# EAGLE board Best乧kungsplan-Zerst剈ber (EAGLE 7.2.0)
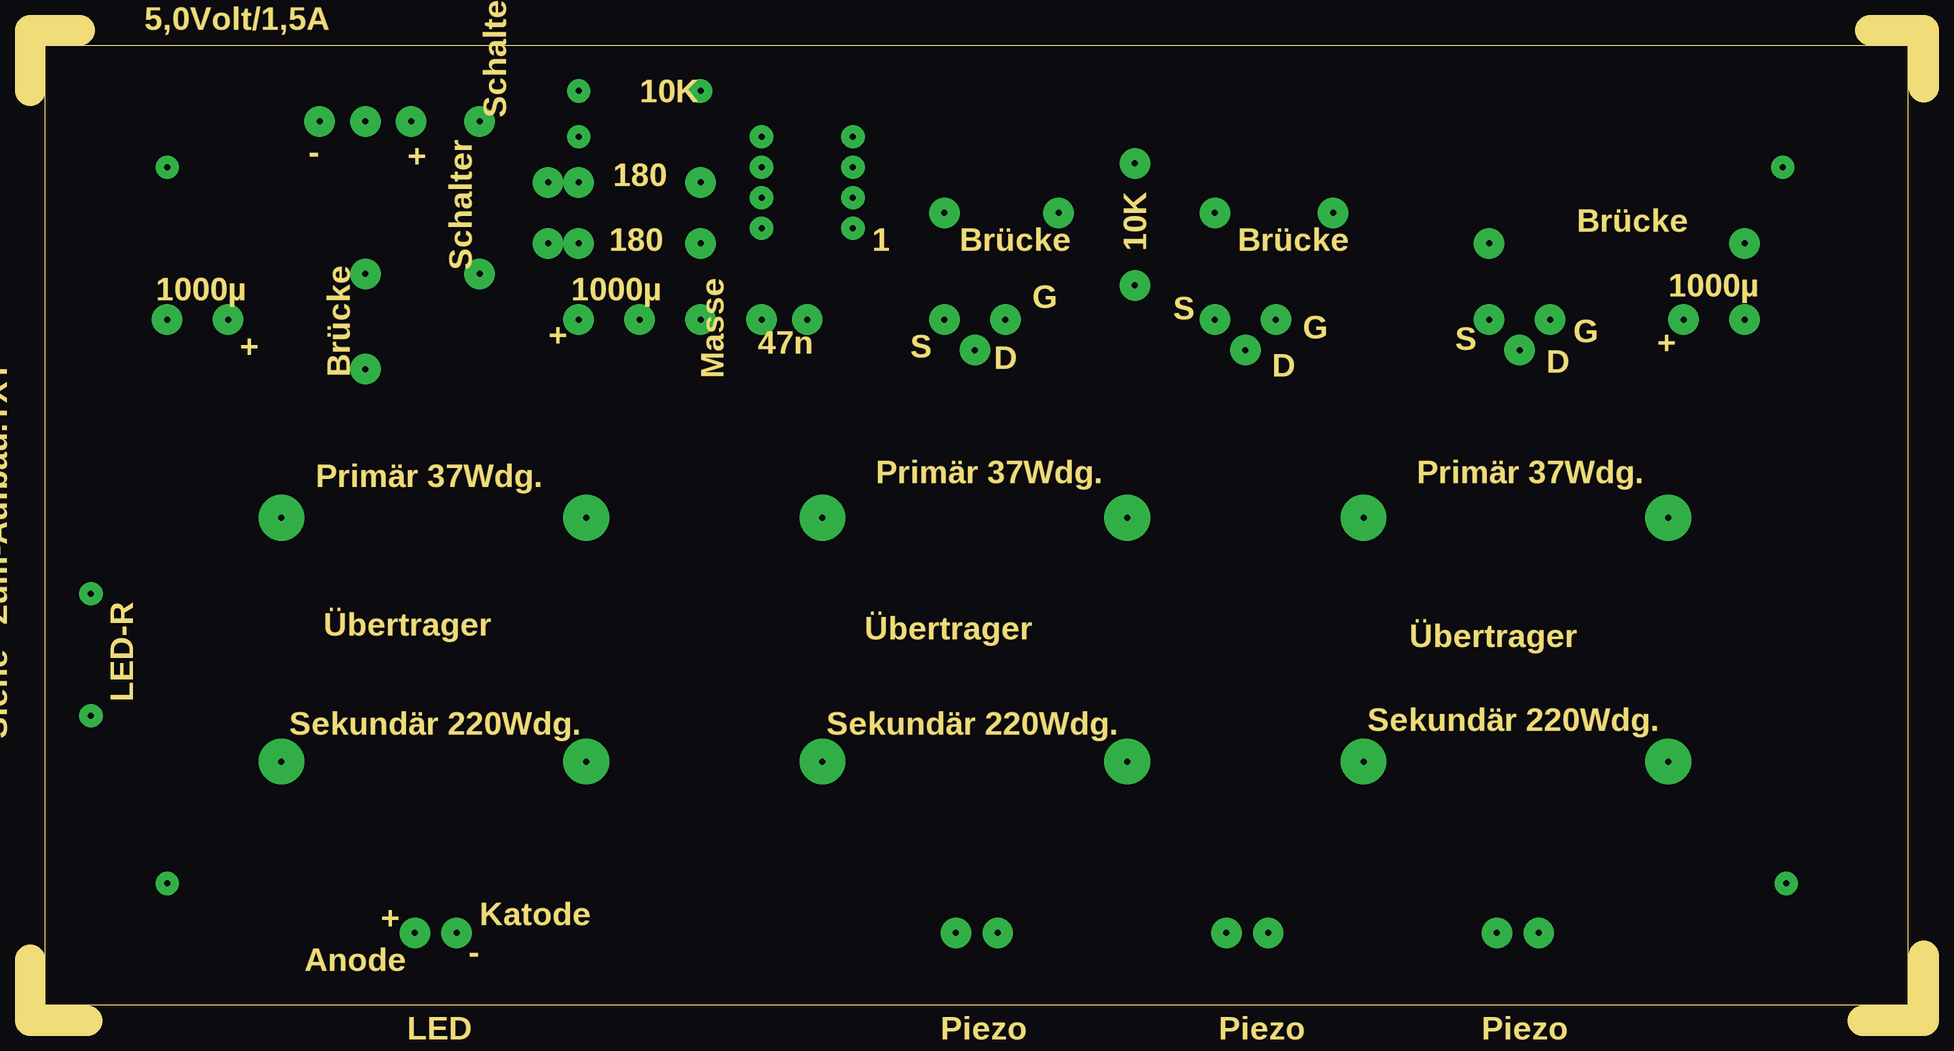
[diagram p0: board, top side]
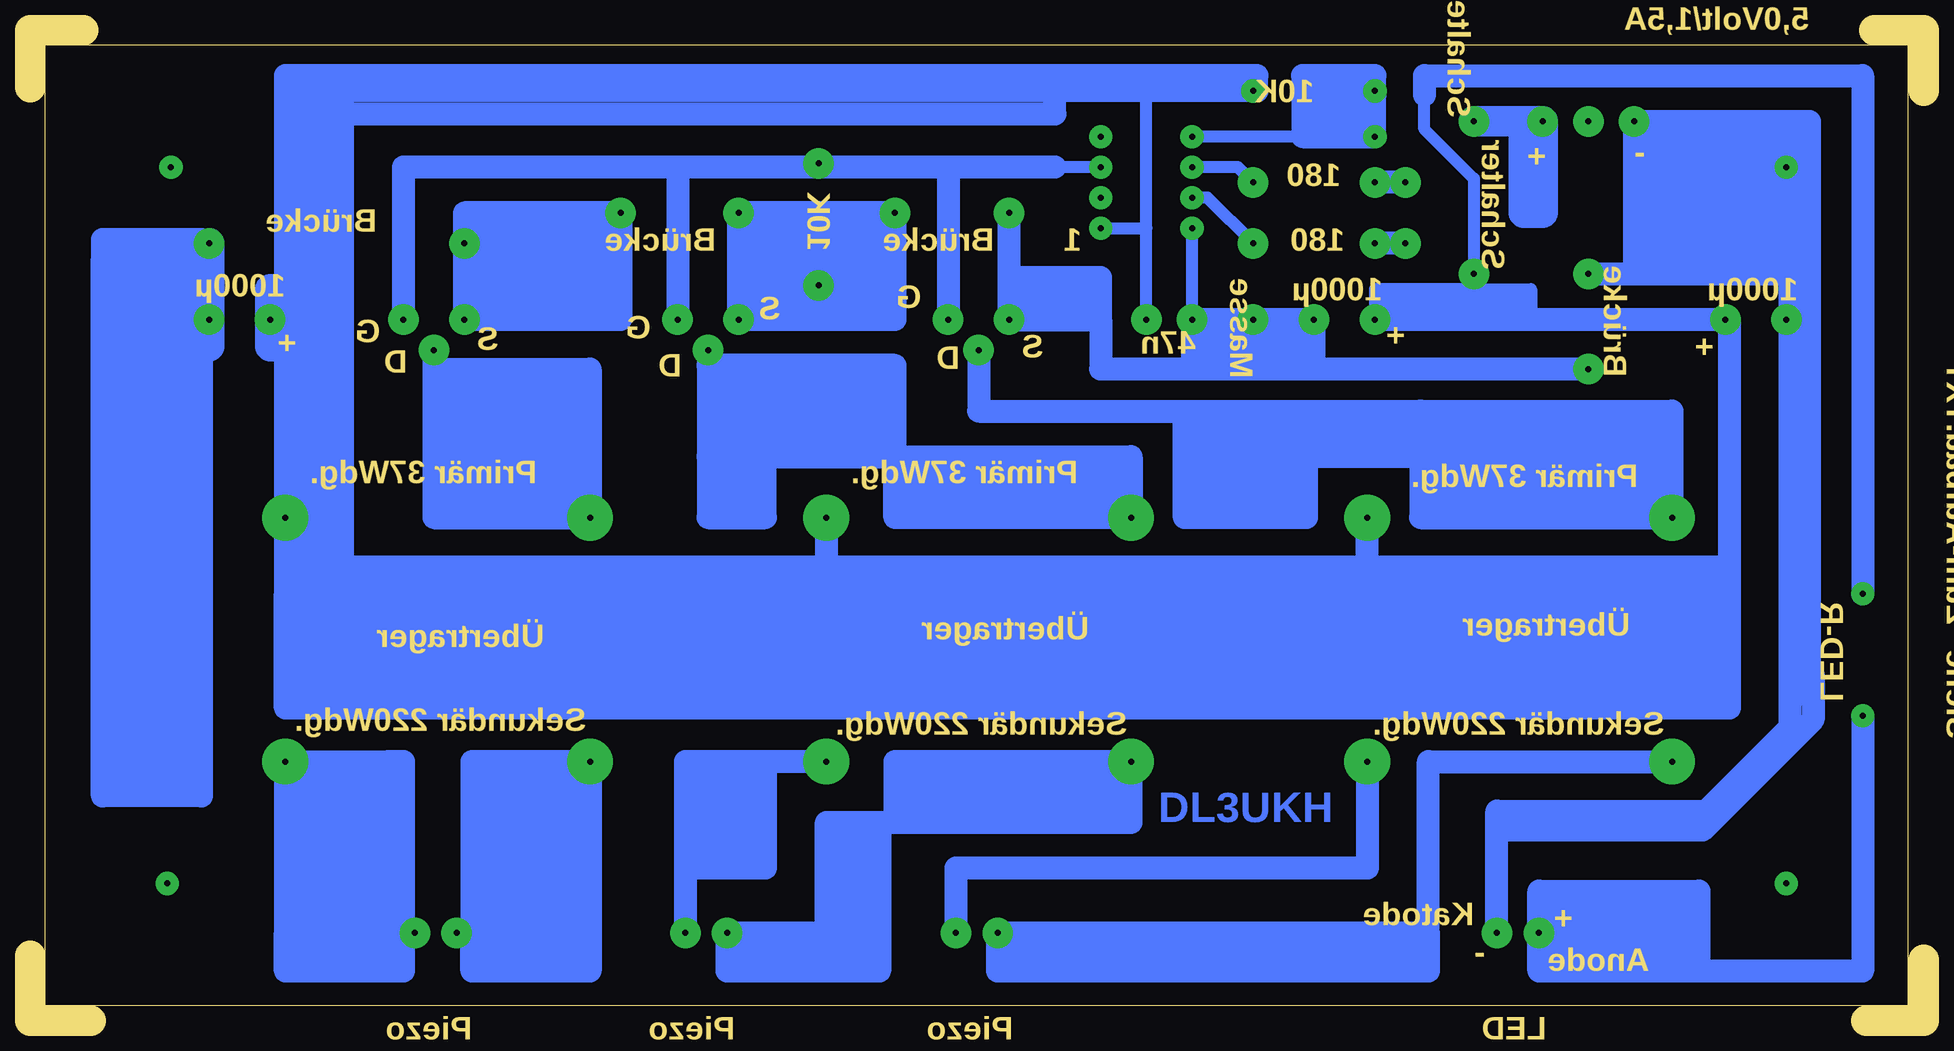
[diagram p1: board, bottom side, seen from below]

Size 157.8 x 82.55 mm. Coordinates in mm from the lower left corner, seen from the top.
Outline: 157.8,5.4 157.8,0.32
Outline: 157.8,0 152.72,0
Outline: 157.8,77.79 157.8,82.55 153.35,82.55
Outline: 0,5.08 0,0 4.76,0
Outline: 4.13,82.55 0,82.55
Outline: 0,77.47 0,82.23
Outline: 156.53,1.27 156.53,81.28 1.27,81.28 1.27,1.27 156.53,1.27
Copper layers (1*16): Top 0.035mm / dielectric 1.5mm / Bottom 0.035mm
Design rules "default": minimum track width 10mil, minimum drill 24mil, track to track 8mil, track to pad 8mil, pad to pad 8mil, via to via 8mil, smd to smd 8mil, copper to edge 40mil, drill to drill 8mil, minimum pad ring 10mil, minimum via ring 8mil, stop-mask expansion 4mil, vias tented up to drill 0mil, thermal gap 10mil

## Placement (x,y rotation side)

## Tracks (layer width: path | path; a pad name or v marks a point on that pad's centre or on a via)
S$1  (via drill 0.5 pad 1.93)
  other vias: 11.43,71.12
S$2  (via drill 0.5 pad 1.93)
  other vias: 11.43,11.43
S$3  (via drill 0.5 pad 1.93)
  other vias: 146.05,71.12
S$4  (via drill 0.5 pad 1.93)
  other vias: 146.37,11.43
S$5  (via drill 0.5 pad 1.93)
  other vias: 5.08,35.56
S$6  (via drill 0.5 pad 2.54)
  Bottom 1.016: 11.11,61.6 11.43,62.23 14.92,62.23
  Bottom 1.93: v35.56,7.3 35.56,17.46 18.1,17.46 11.11,24.45 11.11,61.6 11.11,62.23 | 27.94,62.23 24.13,62.23 | 24.13,62.23 11.43,62.23 | 14.92,74.93 v24.13,74.93 24.13,62.23 | 14.92,74.93 14.92,62.23 | 14.92,74.93 9.53,74.93 9.53,61.91 | 9.53,61.91 14.29,62.87 14.61,62.23 | 9.53,61.91 9.53,26.99
S$7  (via drill 0.5 pad 2.54)
  Bottom 1.016: v60.96,58.42 60.96,66.04 | 55.88,54.61 55.88,53.98 | 60.96,53.98 60.96,54.61 | 55.88,53.98 60.96,53.98 | 50.8,53.98 55.88,53.98 | 50.8,54.93 50.8,53.98 | 27.62,53.98 50.8,53.98 | 60.96,53.98 68.58,53.98 68.58,54.29
  Bottom 1.93: v55.88,58.42 55.88,54.61 | 50.8,54.93 v50.8,58.42 v60.96,58.42 60.96,54.61 | 76.2,61.91 v76.2,58.42 68.58,58.42 | 76.2,61.91 v76.2,67.31 | 68.58,58.42 68.58,54.29 v27.94,54.29 | 68.58,58.42 68.58,61.91 76.2,61.91
S$8  (via drill 0.5 pad 2.54)
  Bottom 1.93: v43.18,69.85 v45.72,69.85
S$9  (via drill 0.5 pad 2.54)
  Bottom 1.93: v43.18,64.77 v45.72,64.77
S$10  (via drill 0.5 pad 2.54, 0.5 pad 3.81)
  Bottom 1.93: v99.69,7.3 91.44,7.3 | 91.44,7.3 91.44,16.51 86.99,16.51 | 86.99,16.51 85.72,16.51 | 85.72,16.51 66.04,16.51 v66.04,21.59 85.72,21.59 85.72,16.51 | 91.44,7.3 91.44,4.13 | 91.44,4.13 92.08,4.13 99.69,4.13 99.69,6.98 | 86.99,16.51 86.99,4.13 91.44,4.13
S$11  (via drill 0.5 pad 2.54)
  Bottom 1.93: v85.72,67.31 85.72,58.42 v98.74,58.42 v98.74,67.31 v85.72,67.31
S$12  (via drill 0.5 pad 2.54, 0.5 pad 3.81)
  Bottom 1.93: v78.74,55.88 78.74,50.8 41.91,50.8 | 41.91,50.8 20.95,50.8 v20.95,41.91 41.91,41.91 41.91,46.99 | 41.91,50.8 41.91,46.99 | 41.91,46.99 51.44,46.99 | 51.44,46.99 61.6,46.99 | 61.6,46.99 61.6,47.31 61.6,50.48 | 51.44,46.99 51.44,41.91 61.6,41.91 61.6,46.99
S$13  (via drill 0.5 pad 2.54)
  Bottom 1.93: 33.02,74.93 33.34,74.93
  Bottom 2.54: v37.47,74.93 33.34,74.93 33.34,67.31 31.75,67.31 v31.75,74.93 33.02,74.93
S$14  (via drill 0.5 pad 2.54, 0.5 pad 3.81)
  Bottom 1.93: v46.36,21.59 46.36,12.7 80.64,12.7 v80.64,7.3
S$15  (via drill 0.5 pad 2.54)
  other vias: 27.94,62.23
S$16  (via drill 0.5 pad 2.54)
  Bottom 1.93: v108.58,67.31 108.58,58.42 v121.6,58.42 v121.6,64.77 121.6,67.31 v108.58,67.31
S$17  (via drill 0.5 pad 2.54, 0.5 pad 3.81)
  Bottom 1.93: 41.28,7.3 v77.15,7.3 77.15,4.13 41.28,4.13 41.28,7.3 | 41.28,7.3 41.28,21.59 v20.95,21.59
S$18  (via drill 0.5 pad 2.54, 0.5 pad 3.81)
  Bottom 1.93: v91.44,21.59 96.52,21.59 | 96.52,21.59 103.19,21.59 v103.19,7.3 | 96.52,21.59 96.52,12.7 102.87,12.7
S$19  (via drill 0.5 pad 2.54)
  other vias: 11.43,58.42
S$20  (via drill 0.5 pad 2.54)
  other vias: 27.94,74.93
S$21  (via drill 0.5 pad 1.93)
  Bottom 1.016: v45.72,77.47 52.07,77.47 52.07,73.66 | 52.07,73.66 v60.96,73.66 | 51.75,73.66 52.07,73.66
  Bottom 1.93: v45.72,77.47 45.72,78.74 51.75,78.74 51.75,73.66 v45.72,73.66 45.72,77.15 v45.72,77.47
S$22  (via drill 0.5 pad 2.54, 0.5 pad 3.81)
  Bottom 1.93: 136.53,7.3 v136.53,21.59 127.95,21.59 | 136.53,7.3 v125.73,7.3 | 126.68,4.13 136.53,4.13 136.53,7.3 | 127.95,21.59 127.95,6.67 | 126.68,21.59 127.95,21.59
S$23  (via drill 0.5 pad 1.93, 0.5 pad 2.54)
  Bottom 1.016: v55.88,69.85 57.15,71.12 v60.96,71.12
S$24  (via drill 0.5 pad 1.93, 0.5 pad 2.54)
  Bottom 1.93: v5.08,25.4 5.08,4.13 18.73,4.13 | 18.73,4.13 32.07,4.13 v32.07,7.3 | v32.07,7.3 18.73,7.3 | 18.73,7.3 18.73,6.98 18.73,4.13 | v32.07,7.3 32.07,10.79 18.73,10.79 18.73,7.3
S$25  (via drill 0.5 pad 2.54)
  other vias: 92.08,71.44
S$26  (via drill 0.5 pad 1.93, 0.5 pad 2.54)
  Bottom 1.016: v55.88,64.77 59.69,68.58 v60.96,68.58
S$27
  Bottom 1.93: 131.45,75.56 72.39,75.56 72.39,77.15
S$28  (via drill 0.5 pad 2.54)
  other vias: 92.08,61.28
S$29  (via drill 0.5 pad 2.54, 0.5 pad 3.81)
  Bottom 1.93: v124.14,55.88 124.14,54.29 | 124.14,54.29 124.14,41.91 v111.12,41.91 111.12,54.29 124.14,54.29
S$30
  Bottom 1.93: 9.21,28.89 9.21,25.08 18.41,15.88 35.24,15.88
S$31
  Bottom 1.93: 143.51,63.5 143.51,18.73 151.77,18.73 151.77,63.18 151.77,63.5 | 151.77,63.5 143.51,63.5 | 143.51,63.5 143.51,65.09 151.77,65.09 151.77,63.5
S$32  (via drill 0.5 pad 2.54, 0.5 pad 3.81)
  Bottom 1.93: v101.28,55.88 101.28,54.61 | 101.28,54.61 101.28,46.99 | 101.28,46.99 85.72,46.99 | 85.72,46.99 66.04,46.99 v66.04,41.91 85.72,41.91 85.72,46.99 | 85.72,46.99 85.72,54.61 101.28,54.61 | 101.28,46.99 101.28,41.91 96.52,41.91 96.52,46.36
S$33  (via drill 0.5 pad 1.93, 0.5 pad 2.54, 0.5 pad 3.81)
  Bottom 1.016: v68.58,66.04 64.77,66.04 | 64.77,66.04 64.77,77.47 | v64.77,58.42 64.77,66.04 | 41.59,77.15 41.59,74.3 37.47,70.17 v37.47,62.23 | v45.72,58.42 45.72,60.96 37.47,60.96 32.7,60.96 32.7,58.74
  Bottom 1.93: 55.56,77.47 55.56,78.74 136.53,78.74 136.53,77.47 | 131.76,77.47 64.77,77.47 v55.88,77.47 | 131.76,77.47 136.53,77.47 | 136.53,35.56 v136.53,41.91 136.53,77.47 | 136.53,35.56 131.76,35.56 | 131.76,35.56 91.44,35.56 | v91.44,41.91 91.44,35.56 | 91.44,35.56 46.36,35.56 | 46.36,35.56 v46.36,41.91 | 16.19,35.56 46.36,35.56 | 16.19,37.78 16.19,58.42 v16.51,58.42 37.47,58.42 | 16.19,37.78 16.19,35.56 | 131.76,77.47 131.76,35.56 | 16.19,37.78 133.03,37.78 133.03,38.1 | 16.19,35.56 16.19,26.04 136.53,26.04 136.53,35.56 | 5.08,35.56 5.08,78.74 41.59,78.74 41.59,77.15 | 37.47,58.42 v45.72,58.42 | v37.47,62.23 37.47,60.96 37.47,58.42
S$34  (via drill 0.5 pad 2.54)
  Bottom 2.54: v137.8,58.42 135.57,58.42 | 135.89,60.96 137.8,60.96 v137.8,58.42 | v137.8,58.42 137.8,56.2 134.94,56.2
S$35  (via drill 0.5 pad 1.93)
  other vias: 60.96,66.04
S$36  (via drill 0.5 pad 2.54)
  Bottom 2.54: 142.88,64.77 v142.88,58.42 142.88,56.2
S$38  (via drill 0.5 pad 2.54, 0.5 pad 3.81)
  Bottom 1.93: 120.97,21.59 v111.12,21.59 111.12,7.3 | 111.12,7.3 v122.24,7.3 | 111.12,7.3 111.12,4.13 120.33,4.13 | 120.33,4.13 120.33,7.62 | 120.33,4.13 120.97,4.13 120.97,7.62
S$39  (via drill 0.5 pad 1.93)
  other vias: 68.58,68.58
S$40  (via drill 0.5 pad 2.54)
  other vias: 142.88,64.77
S$49  (via drill 0.5 pad 1.93, 0.5 pad 2.54)
  Bottom 1.016: v68.58,71.12 72.39,71.12 81.28,71.12
  Bottom 1.93: 81.28,71.12 v81.28,58.42 | 81.28,71.12 82.23,71.12 103.82,71.12 | 103.82,71.12 v103.82,58.42 | 103.82,71.12 126.68,71.12 v126.68,58.42 | 72.39,71.12 81.28,71.12
S$56  (via drill 0.5 pad 1.93)
  other vias: 68.58,73.66
(copper drawn outside any net)
  shapes: Bottom area x32

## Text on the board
Bottom: DL3UKH
Vias: Auf Bestückungsseite gesehen !
Dimension: Taster | Steckernetzteil | 5,0Volt/1,5A | 10K | Schalter | - | + | 180 | Brücke | 180 | 1 | Brücke | 10K | Brücke | Schalter | Masse | 1000µ | 1000µ | 1000µ | G | S | G | + | S | G | + | 47n | S | + | D | D | Brücke | D | Primär 37Wdg. | Primär 37Wdg. | Primär 37Wdg. | LED-R | Übertrager | Übertrager | Übertrager | Sekundär 220Wdg. | Sekundär 220Wdg. | Sekundär 220Wdg. | Siehe "Zum-Aufbau.TXT" | Katode | + | Anode | - | LED | Piezo | Piezo | Piezo | G | S | Siehe "Zum-Aufbau.TXT" | D | 1 stck. Anschluss-Leiste Steckernetzteil 5,0Volt 1,35mm | Die 4 Brücken nicht vergessen ! | 4 stck. Anschluss-Leiste Piezo + LED 1,35mm | Übertrager / Trafo 1,35mm | Mosfet IRF3708 oder IRL2505 1,0mm
tOrigins: PIC12F1840 | 1 | Links oben ist | immer PIN 1 | PIC12F1840 | gn | Duo-LED | rt | IRF 3708 | IRF 3708 | IRF 3708 | gn | rt | gemeinsame Katode | an Masse | IRL2505 | oder | IRF3708 | Leiterplatte: | BOHRUNGEN | 1,5mm dick | alles 0.8mm vorbohren | Cevausit | 4 stck. Befestigungsbohr... 3,2mm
